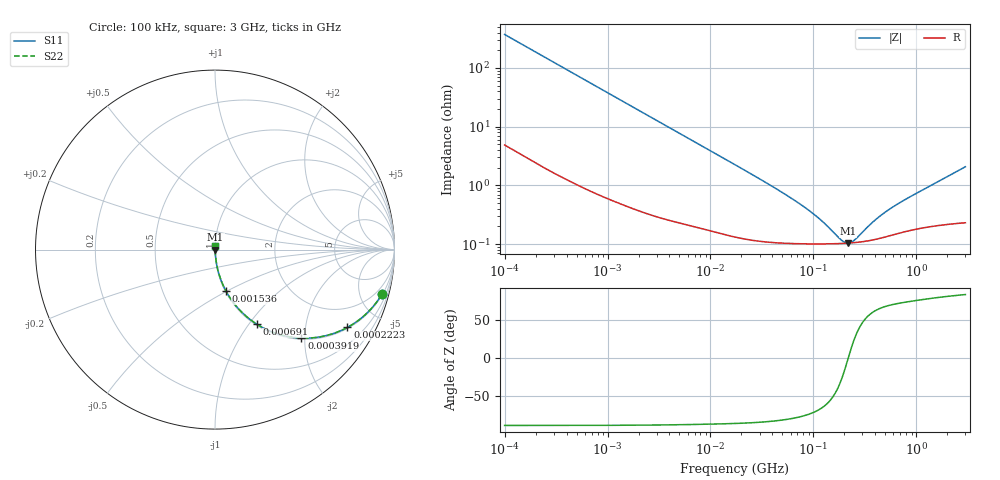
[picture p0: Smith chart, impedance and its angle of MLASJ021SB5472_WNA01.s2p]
! MLASJ021SB5472_WNA01  S-PARAMETER MODEL  ( Standard Model )
! Model Generated by TAIYO YUDEN Corporation (http://www.ty-top.com)
! Version 1.0
! TAIYO YUDEN Control No. 220901
! Copyright(c) 2022 TAIYO YUDEN CO.,LTD. All Rights Reserved.
! Product Description (link to TY-COMPAS)
! https://ds.yuden.co.jp/TYCOMPAS/or/detail?pn=MLASJ021SB5472KWNA01&u=M
! Products Name : Multilayer Ceramic Capacitors
! Characteristics :
!  Capacitance : 4700 [pF] , Rated Voltage : 6.3 [V] , TCC : X5R
!  Case Size : 0.25 x 0.125 / 0.0098 x 0.0049 [mm/inch] , Thickness : 0.125 / 0.0049 [mm/inch]
!  (Conditions: Temperature = 25 [degC] , DC Bias Voltage = 0 [V])
! External Node Assignments :
!  1  o---| |---o  2
! GND o---------o GND
! Frequency Range : 100kHz  -  3GHz  [ 401 STEP ]
# MHZ S RI R 50
! Freq[MHz].  S11 Real  S11 Imag  S21 Real  S21 Imag  S12 Real  S12 Imag  S22 Real  S22 Imag
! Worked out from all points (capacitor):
!   401 points, 100 kHz to 3 GHz, reference 50 ohm
!   read as one part in series: C = 4.25 nF near 105.3 kHz
!   lowest |Z| = 104 mohm at 216.5 MHz (marker M1)
!   series resonance near 218.5 MHz, so ESL is about 120 pH
!   S11 on the Smith chart (normalised r, x): 100 kHz: 1.10, -7.46; 222.3 kHz: 1.04, -3.38; 391.9 kHz: 1.03, -1.93; 691 kHz: 1.02, -1.10; 1.536 MHz: 1.01, -0.50; 3 GHz: 1.00, +0.04
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0.1  0.9302 -0.2483  0.0698 0.2483  0.0698 0.2483  0.9302 -0.2483
0.151038  0.857 -0.3436  0.143 0.3436  0.143 0.3436  0.857 -0.3436
0.222319  0.7381 -0.4333  0.2619 0.4333  0.2619 0.4333  0.7381 -0.4333
0.302894  0.606 -0.4822  0.394 0.4822  0.394 0.4822  0.606 -0.4822
0.391939  0.4813 -0.4931  0.5187 0.4931  0.5187 0.4931  0.4813 -0.4931
0.562235  0.3141 -0.4573  0.6859 0.4573  0.6859 0.4573  0.3141 -0.4573
0.690972  0.2345 -0.4165  0.7655 0.4165  0.7655 0.4165  0.2345 -0.4165
1.017073  0.1264 -0.3245  0.8736 0.3245  0.8736 0.3245  0.1264 -0.3245
1.536162  0.0617 -0.2319  0.9383 0.2319  0.9383 0.2319  0.0617 -0.2319
3.161081  0.0172 -0.1189  0.9828 0.1189  0.9828 0.1189  0.0172 -0.1189
6.674626  0.00534 -0.0575  0.9947 0.0575  0.9947 0.0575  0.00534 -0.0575
17.7727  0.00178 -0.0219  0.9982 0.0219  0.9982 0.0219  0.00178 -0.0219
52.46276  0.00108 -0.00709  0.9989 0.00709  0.9989 0.00709  0.00108 -0.00709
97.38194  0.00102 -0.00325  0.999 0.00325  0.999 0.00325  0.00102 -0.00325
126.0104  0.00101 -0.00209  0.999 0.00209  0.999 0.00209  0.00101 -0.00209
185.4806  0.00102 -0.000596  0.999 0.000596  0.999 0.000596  0.00102 -0.000596
216.4987  0.00104 -3.35e-05  0.999 3.35e-05  0.999 3.35e-05  0.00104 -3.35e-05
252.704  0.00106 0.000527  0.9989 -0.000527  0.9989 -0.000527  0.00106 0.000527
381.6779  0.00118 0.0021  0.9988 -0.0021  0.9988 -0.0021  0.00118 0.0021
547.5153  0.00139 0.00366  0.9986 -0.00366  0.9986 -0.00366  0.00139 0.00366
893.4279  0.00176 0.00632  0.9982 -0.00632  0.9982 -0.00632  0.00176 0.00632
3000  0.00273 0.0206  0.9973 -0.0206  0.9973 -0.0206  0.00273 0.0206
